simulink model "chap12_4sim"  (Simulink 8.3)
settings: Solver=ode45  StartTime=0.0  StopTime=10

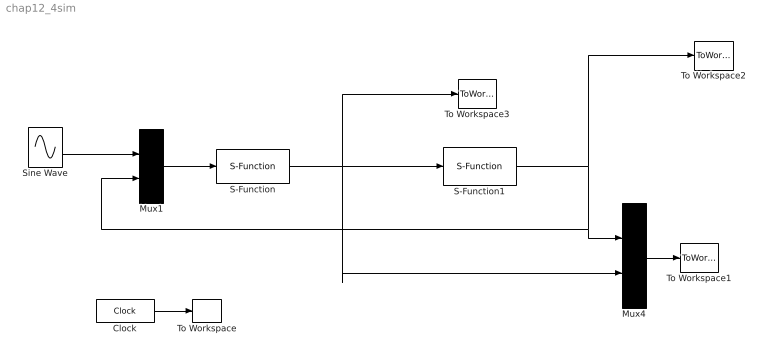
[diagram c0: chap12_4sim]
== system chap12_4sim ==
  Clock : Clock
  Mux1 : Mux  Inputs=2
  Mux4 : Mux  Inputs=2
  S-Function : S-Function  FunctionName=chap12_4ctrl  EnableBusSupport=off
  S-Function1 : S-Function  FunctionName=chap12_4plant  EnableBusSupport=off
  Sine Wave : Sin  SampleTime=0
  To Workspace : ToWorkspace  VariableName=t  SampleTime=-1
  To Workspace1 : ToWorkspace  VariableName=p  SampleTime=-1
  To Workspace2 : ToWorkspace  VariableName=y  SampleTime=-1
  To Workspace3 : ToWorkspace  VariableName=ut  SampleTime=-1
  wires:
  Clock/1 -> To Workspace/1
  Sine Wave/1 -> Mux1/1
  Mux1/1 -> S-Function/1
  S-Function1/1 -> To Workspace2/1, Mux1/2, Mux4/1
  Mux4/1 -> To Workspace1/1
  S-Function/1 -> Mux4/2, S-Function1/1, To Workspace3/1
